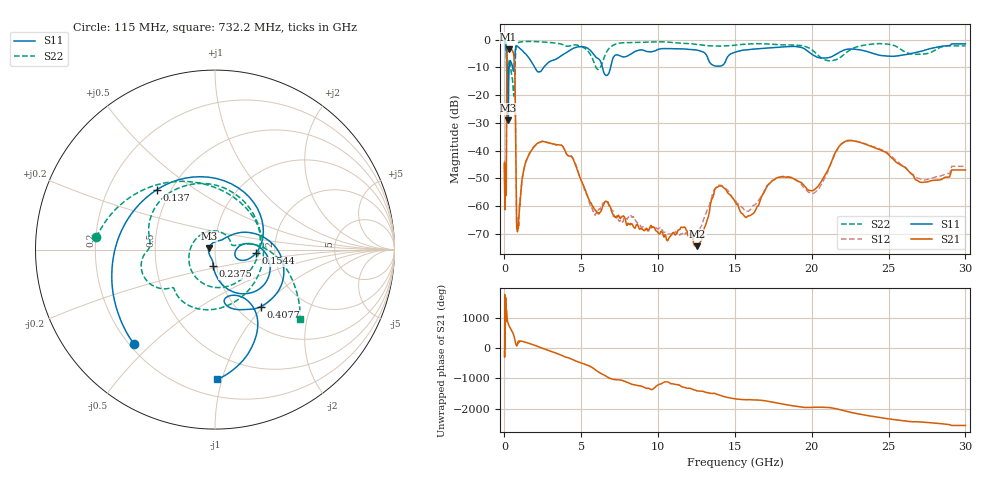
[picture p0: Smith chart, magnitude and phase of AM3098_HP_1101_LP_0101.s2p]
! Date/Time: Thu, Feb 28, 2019 8:45 AM
! Network Analyzer: Agilent Technologies E8364B Rev: A.07.50.67
! Sweep from 0.010 to 30.000 GHz, 1601 Points, Sweep Type: LOG
! Power Supply: 5.022 V, 0.002 A
# Hz S DB R 50
!freq MagS11 AngS11 MagS21 AngS21 MagS12 AngS12 MagS22 AngS22
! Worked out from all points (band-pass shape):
!   1601 points, 10 MHz to 30 GHz, reference 50 ohm
!   highest |S21| = -3.42 dB at 266.5 MHz (marker M1); lowest = -74.4 dB at 12.56 GHz (marker M2)
!   |S21| within 3 dB of the highest: 158.7 MHz to 623.9 MHz (465.2 MHz wide, 119 % of centre)
!   lowest |S11| = -29.1 dB at 249.7 MHz (marker M3), VSWR 1.07, Z = 46.7 + j0.891 ohm
!   |S11| at or under -10 dB: 207.2 MHz to 303.6 MHz (96.34 MHz wide, 37.7 % of centre); 1.975 GHz to 2.551 GHz (576 MHz wide, 25.4 % of centre); 6.371 GHz to 6.908 GHz (537 MHz wide, 8.09 % of centre)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
!   |S22| runs from -20.4 to -0.6 dB; largest |S21 - S12| = 0.011
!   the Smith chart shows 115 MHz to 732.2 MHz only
!   S11 on the Smith chart (normalised r, x): 115 MHz: 0.22, -0.44; 137 MHz: 0.42, +0.36; 154.4 MHz: 1.59, -0.07; 237.5 MHz: 0.96, -0.18; 407.7 MHz: 1.27, -0.97; 732.2 MHz: 0.32, -0.97
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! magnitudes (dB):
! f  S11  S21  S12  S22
! 10 MHz  -0.4  -44.6  -44.3  -0.6
! 38.04 MHz  -0.3  -57.1  -57.9  -0.7
! 115 MHz  -3.2  -55.5  -53.5  -3.6
! 137 MHz  -6.7  -24.6  -24.8  -11.0
! 144.7 MHz  -8.7  -14.2  -14.2  -10.5
! 154.4 MHz  -12.8  -7.6  -7.6  -9.4
! 237.5 MHz  -20.6  -3.5  -3.5  -8.6
! 249.7 MHz  -29.1  -3.5  -3.4  -8.8
! 266.5 MHz  -18.8  -3.4  -3.4  -8.7
! 407.7 MHz  -7.8  -3.6  -3.6  -10.1
! 550.5 MHz  -10.7  -4.4  -4.3  -16.9
! 662.4 MHz  -6.6  -10.1  -10.1  -14.9
! 732.2 MHz  -2.8  -37.2  -37.6  -4.2
! 833.9 MHz  -2.4  -67.7  -66.5  -1.4
! 2.084 GHz  -11.1  -37.6  -37.9  -0.7
! 3.76 GHz  -5.6  -38.2  -38.3  -1.7
! 7.926 GHz  -6.1  -66.3  -64.6  -1.1
! 12.56 GHz  -3.8  -74.4  -69.5  -1.8
! 13.95 GHz  -9.6  -52.7  -52.4  -2.3
! 15.97 GHz  -3.6  -63.4  -61.4  -1.5
! 22.56 GHz  -3.4  -36.3  -36.4  -3.5
! 30 GHz  -1.5  -47.0  -45.6  -2.3
